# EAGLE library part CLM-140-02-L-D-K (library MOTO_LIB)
MICRO SOCKET, 1.0MM pitch, SMD, 2X40WAY, Female
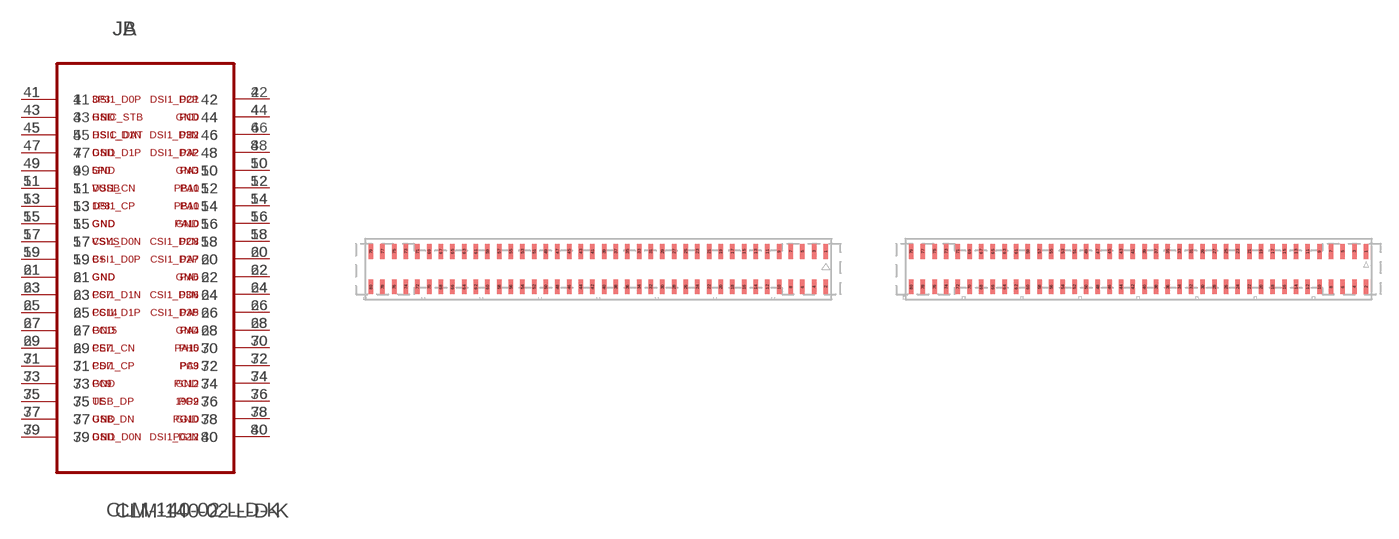
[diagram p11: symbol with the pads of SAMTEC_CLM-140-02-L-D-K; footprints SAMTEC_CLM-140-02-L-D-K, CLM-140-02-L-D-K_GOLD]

Designator prefix J; gates A=CLM-140-02-L-D-K_A B=CLM-140-02-L-D-K_B

## CLM-140-02-L-D-KSOLDER (MPN: CLM-140-02-L-D-K; SUPPLIER: SAMTEC)  [SAMTEC_CLM-140-02-L-D-K]
1  A:1  pas
2  A:2  pas
3  A:3  pas
4  A:4  pas
5  A:5  pas
6  A:6  pas
7  A:7  pas
8  A:8  pas
9  A:9  pas
10  A:10  pas
11  A:11  pas
12  A:12  pas
13  A:13  pas
14  A:14  pas
15  A:15  pas
16  A:16  pas
17  A:17  pas
18  A:18  pas
19  A:19  pas
20  A:20  pas
21  A:21  pas
22  A:22  pas
23  A:23  pas
24  A:24  pas
25  A:25  pas
26  A:26  pas
27  A:27  pas
28  A:28  pas
29  A:29  pas
30  A:30  pas
31  A:31  pas
32  A:32  pas
33  A:33  pas
34  A:34  pas
35  A:35  pas
36  A:36  pas
37  A:37  pas
38  A:38  pas
39  A:39  pas
40  A:40  pas
41  B:41  pas
42  B:42  pas
43  B:43  pas
44  B:44  pas
45  B:45  pas
46  B:46  pas
47  B:47  pas
48  B:48  pas
49  B:49  pas
50  B:50  pas
51  B:51  pas
52  B:52  pas
53  B:53  pas
54  B:54  pas
55  B:55  pas
56  B:56  pas
57  B:57  pas
58  B:58  pas
59  B:59  pas
60  B:60  pas
61  B:61  pas
62  B:62  pas
63  B:63  pas
64  B:64  pas
65  B:65  pas
66  B:66  pas
67  B:67  pas
68  B:68  pas
69  B:69  pas
70  B:70  pas
71  B:71  pas
72  B:72  pas
73  B:73  pas
74  B:74  pas
75  B:75  pas
76  B:76  pas
77  B:77  pas
78  B:78  pas
79  B:79  pas
80  B:80  pas

## CLM-140-02-L-D-KGOLD (MPN: CLM-140-02-L-D-K; SUPPLIER: SAMTEC)  [CLM-140-02-L-D-K_GOLD]
Pads as for SAMTEC_CLM-140-02-L-D-K

## Footprint SAMTEC_CLM-140-02-L-D-K (pad centres in mm)
smd 0.38 x 1.27: 1 19.5,1.52; 2 19.5,-1.52; 3 18.5,1.52; 4 18.5,-1.52; 5 17.5,1.52; 6 17.5,-1.52; 7 16.5,1.52; 8 16.5,-1.52; 9 15.5,1.52; 10 15.5,-1.52; 11 14.5,1.52; 12 14.5,-1.52; 13 13.5,1.52; 14 13.5,-1.52; 15 12.5,1.52; 16 12.5,-1.52; 17 11.5,1.52; 18 11.5,-1.52; 19 10.5,1.52; 20 10.5,-1.52; 21 9.5,1.52; 22 9.5,-1.52; 23 8.5,1.52; 24 8.5,-1.52; 25 7.5,1.52; 26 7.5,-1.52; 27 6.5,1.52; 28 6.5,-1.52; 29 5.5,1.52; 30 5.5,-1.52; 31 4.5,1.52; 32 4.5,-1.52; 33 3.5,1.52; 34 3.5,-1.52; 35 2.5,1.52; 36 2.5,-1.52; 37 1.5,1.52; 38 1.5,-1.52; 39 0.5,1.52; 40 0.5,-1.52; 41 -0.5,1.52; 42 -0.5,-1.52; 43 -1.5,1.52; 44 -1.5,-1.52; 45 -2.5,1.52; 46 -2.5,-1.52; 47 -3.5,1.52; 48 -3.5,-1.52; 49 -4.5,1.52; 50 -4.5,-1.52; 51 -5.5,1.52; 52 -5.5,-1.52; 53 -6.5,1.52; 54 -6.5,-1.52; 55 -7.5,1.52; 56 -7.5,-1.52; 57 -8.5,1.52; 58 -8.5,-1.52; 59 -9.5,1.52; 60 -9.5,-1.52; 61 -10.5,1.52; 62 -10.5,-1.52; 63 -11.5,1.52; 64 -11.5,-1.52; 65 -12.5,1.52; 66 -12.5,-1.52; 67 -13.5,1.52; 68 -13.5,-1.52; 69 -14.5,1.52; 70 -14.5,-1.52; 71 -15.5,1.52; 72 -15.5,-1.52; 73 -16.5,1.52; 74 -16.5,-1.52; 75 -17.5,1.52; 76 -17.5,-1.52; 77 -18.5,1.52; 78 -18.5,-1.52; 79 -19.5,1.52; 80 -19.5,-1.52

## Footprint CLM-140-02-L-D-K_GOLD (pad centres in mm)
smd 0.38 x 1.27: 1 19.5,1.52; 2 19.5,-1.52; 3 18.5,1.52; 4 18.5,-1.52; 5 17.5,1.52; 6 17.5,-1.52; 7 16.5,1.52; 8 16.5,-1.52; 9 15.5,1.52; 10 15.5,-1.52; 11 14.5,1.52; 12 14.5,-1.52; 13 13.5,1.52; 14 13.5,-1.52; 15 12.5,1.52; 16 12.5,-1.52; 17 11.5,1.52; 18 11.5,-1.52; 19 10.5,1.52; 20 10.5,-1.52; 21 9.5,1.52; 22 9.5,-1.52; 23 8.5,1.52; 24 8.5,-1.52; 25 7.5,1.52; 26 7.5,-1.52; 27 6.5,1.52; 28 6.5,-1.52; 29 5.5,1.52; 30 5.5,-1.52; 31 4.5,1.52; 32 4.5,-1.52; 33 3.5,1.52; 34 3.5,-1.52; 35 2.5,1.52; 36 2.5,-1.52; 37 1.5,1.52; 38 1.5,-1.52; 39 0.5,1.52; 40 0.5,-1.52; 41 -0.5,1.52; 42 -0.5,-1.52; 43 -1.5,1.52; 44 -1.5,-1.52; 45 -2.5,1.52; 46 -2.5,-1.52; 47 -3.5,1.52; 48 -3.5,-1.52; 49 -4.5,1.52; 50 -4.5,-1.52; 51 -5.5,1.52; 52 -5.5,-1.52; 53 -6.5,1.52; 54 -6.5,-1.52; 55 -7.5,1.52; 56 -7.5,-1.52; 57 -8.5,1.52; 58 -8.5,-1.52; 59 -9.5,1.52; 60 -9.5,-1.52; 61 -10.5,1.52; 62 -10.5,-1.52; 63 -11.5,1.52; 64 -11.5,-1.52; 65 -12.5,1.52; 66 -12.5,-1.52; 67 -13.5,1.52; 68 -13.5,-1.52; 69 -14.5,1.52; 70 -14.5,-1.52; 71 -15.5,1.52; 72 -15.5,-1.52; 73 -16.5,1.52; 74 -16.5,-1.52; 75 -17.5,1.52; 76 -17.5,-1.52; 77 -18.5,1.52; 78 -18.5,-1.52; 79 -19.5,1.52; 80 -19.5,-1.52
